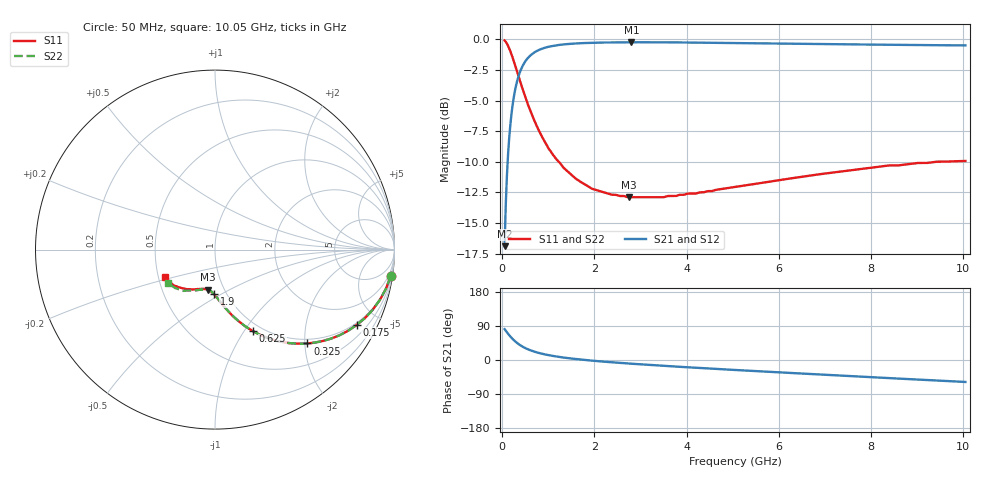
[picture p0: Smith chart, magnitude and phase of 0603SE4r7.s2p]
! AVX Thin Film Operation		Date: August 2001
! Description: Accu-P® Series, Thin Film, SMD, RF Capacitor
! Part Number: 06035J4R7ABT
! 50 MHz  -  10.05 GHz
! Serial Measurements
# mhz S db R 50
!	S11		S21		S12		S22
!	dB	Phase	dB	Phase	dB	Phase	dB	Phase
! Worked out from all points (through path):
!   401 points, 50 MHz to 10.05 GHz, reference 50 ohm
!   highest |S21| = -0.24 dB at 2.8 GHz (marker M1); lowest = -16.9 dB at 50 MHz (marker M2)
!   group delay of S21, straight-line fit = 24 ps
!   lowest |S11| = -12.9 dB at 2.75 GHz (marker M3), VSWR 1.59, Z = 42.1 - j19.8 ohm
!   |S11| at or under -10 dB: 1.225 GHz to 9.425 GHz (8.2 GHz wide, 154 % of centre)
!   |S22| runs from -12.9 to -0.1 dB; largest |S21 - S12| = 0
!   S11 on the Smith chart (normalised r, x): 50 MHz: 1, -13; 175 MHz: 0.91, -3.80; 325 MHz: 0.91, -2.06; 625 MHz: 0.90, -1.10; 1.9 GHz: 0.88, -0.46; 10.05 GHz: 0.54, -0.19
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50  -0.09 -8.6  -16.90 81.4  -16.90 81.4  -0.09 -8.6
75  -0.20 -12.8  -13.51 77.2  -13.51 77.2  -0.20 -12.8
125  -0.53 -20.8  -9.40 69.1  -9.40 69.1  -0.53 -20.8
175  -0.98 -28.1  -6.97 62.0  -6.97 62.0  -0.98 -28.1
250  -1.79 -37.6  -4.72 52.4  -4.72 52.4  -1.79 -37.6
325  -2.69 -45.4  -3.36 44.6  -3.36 44.6  -2.69 -45.4
400  -3.58 -51.8  -2.50 38.2  -2.50 38.2  -3.58 -51.8
475  -4.45 -57.1  -1.94 32.9  -1.94 32.9  -4.45 -57.1
625  -5.99 -65.0  -1.26 25.0  -1.26 25.0  -5.99 -65.0
800  -7.50 -71.6  -0.86 18.4  -0.86 18.4  -7.49 -71.5
1025  -9.03 -77.7  -0.59 12.3  -0.59 12.3  -9.03 -77.6
1350  -10.57 -83.9  -0.40 6.1  -0.40 6.1  -10.57 -83.7
1725  -11.70 -89.2  -0.31 0.9  -0.31 0.9  -11.70 -88.8
1900  -12.10 -91.2  -0.28 -1.2  -0.28 -1.2  -12.05 -90.8
2325  -12.64 -95.7  -0.25 -5.5  -0.25 -5.5  -12.64 -95.0
2750  -12.90 -99.5  -0.24 -9.4  -0.24 -9.4  -12.90 -98.7
2800  -12.90 -99.9  -0.24 -9.8  -0.24 -9.8  -12.90 -99.1
3400  -12.90 -104.8  -0.24 -14.6  -0.24 -14.6  -12.90 -103.8
5050  -12.06 -117.4  -0.29 -26.3  -0.29 -26.3  -12.06 -114.4
6725  -11.10 -129.0  -0.37 -37.1  -0.37 -37.1  -11.10 -125.0
8400  -10.30 -140.1  -0.44 -47.8  -0.44 -47.8  -10.29 -135.1
10050  -9.94 -150.8  -0.49 -58.0  -0.49 -58.0  -9.90 -144.6
